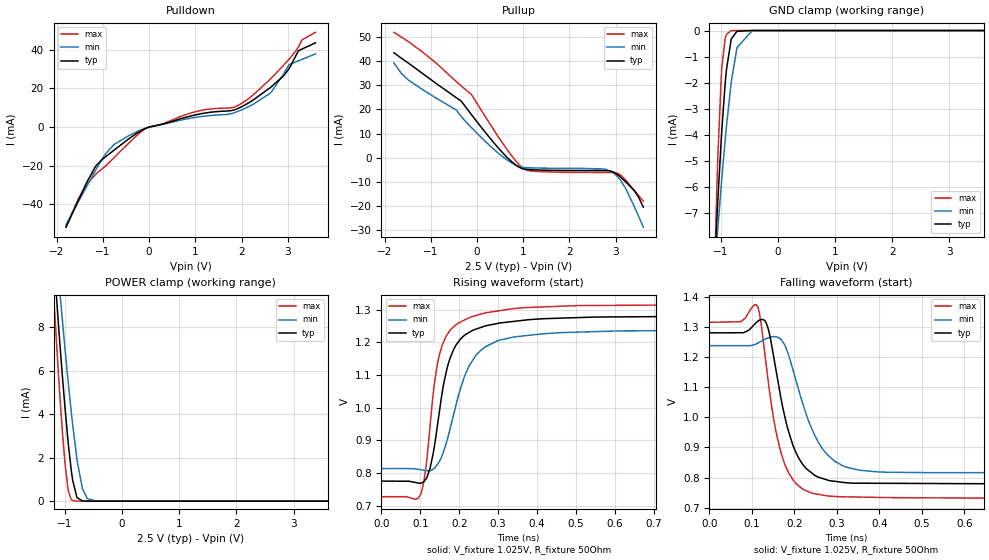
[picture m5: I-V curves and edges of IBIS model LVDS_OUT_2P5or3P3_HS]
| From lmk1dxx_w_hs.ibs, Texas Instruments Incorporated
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|   LVDS_OUT_2P5or3P3_HS Model
[Model]   LVDS_OUT_2P5or3P3_HS
Model_type   Output
Polarity   Non-Inverting
Vmeas = 1.025
Vref = 1.025
Cref = 2pF
Rref = 50
|   typ   min   max
C_comp   0.89pF   0.82pF   0.98pF
[Rac]   50   NA   NA
[Cac]   2p   NA   NA
[Voltage Range]   2.5   2.375   2.625
[Temperature Range]   45   150   -40
[Pullup Reference]   2.5   2.375   2.625
[Pulldown Reference]   0   0   0
[Power Clamp Reference]   2.5   2.375   2.625
[GND Clamp Reference]   0   0   0
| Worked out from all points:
|   slope of the pulldown table from 0 to 0.375 V, typ, clamps not added: 182 ohm
|   slope of the pullup table from 0 to 0.375 V, typ, clamps not added: 41.9 ohm
|   GND clamp passes 1 mA (typ) near -0.87 V on its own axis
|   POWER clamp passes 1 mA (typ) near -0.87 V on its own axis
|   falling waveform, V_fixture 1.025V, R_fixture 50Ohm: 20-80 % time 52.4ps typ, 67.7ps min, 45.7ps max; typ from 1.28 V to 0.775 V
|   rising waveform, V_fixture 1.025V, R_fixture 50Ohm: 20-80 % time 51ps typ, 70.8ps min, 41.6ps max; typ from 0.775 V to 1.28 V
[Pulldown]
|   Voltage   I(typ)   I(min)   I(max)
-1.8V     -51.71mA   -50.46mA   -51.59mA
-1.532V   -37.86mA   -38.59mA   -36.99mA
-1.175V   -20.92mA   -22.95mA   -24.82mA
-763.7mV  -11.99mA   -9.059mA   -15.94mA
-42.3mV   -331.8uA   -287uA     -398.5uA
1.007V    6.329mA    5.035mA    7.964mA
2.004V    10.56mA    8.93mA     12.31mA
2.61V     20.21mA    17.33mA    24.49mA
3.028V    30.21mA    32.21mA    35.05mA
3.232V    39.43mA    34.24mA    41.46mA
3.307V    40.33mA    34.98mA    45.04mA
3.6V      43.54mA    37.85mA    48.98mA
[GND Clamp]
|   Voltage   I(typ)   I(min)   I(max)
-1.8V     -47.22mA   -32.28mA   -90.43mA
-1.103V   -8.782mA   -9.069mA   -8.722mA
-1.072V   -7.372mA   -8.153mA   -6.225mA
-1.053V   -6.556mA   -7.61mA    -4.893mA
-988.9mV  -4.055mA   -5.855mA   -1.636mA
-982.4mV  -3.827mA   -5.684mA   -1.42mA
-922.5mV  -2.008mA   -4.177mA   -294.7uA
-899.8mV  -1.477mA   -3.648mA   -144.9uA
-818.3mV  -346uA     -1.998mA   -5.222uA
-717.3mV  -29.3uA    -659.5uA   -36.6nA
-450mV    -2.386nA   -3.724uA   -6.465pA
3.6V      0A         0A         0A
[Pullup]
|   Voltage   I(typ)   I(min)   I(max)
-1.8V     43.62mA    39.39mA    52.14mA
-1.481V   39.25mA    32.16mA    48.18mA
-450mV    24.91mA    19.81mA    31.63mA
-347.4mV  23.58mA    17.22mA    29.89mA
-122.2mV  17.9mA     12.47mA    26.28mA
581.9mV   1.41mA     -27.44uA   5.168mA
1.007V    -4.767mA   -4.124mA   -4.59mA
1.39V     -5.227mA   -4.407mA   -5.881mA
2.89V     -5.648mA   -5.748mA   -6.237mA
3.15V     -8.931mA   -10.75mA   -8.061mA
3.399V    -13.74mA   -20.23mA   -13.55mA
3.6V      -20.68mA   -29.01mA   -18.2mA
[POWER Clamp]
|   Voltage   I(typ)   I(min)   I(max)
-1.8V     35.35mA    33.02mA    38.41mA
-1.235V   12.58mA    14.14mA    11.07mA
-1.108V   7.901mA    10.18mA    5.58mA
-1.068V   6.535mA    8.999mA    4.045mA
-1V       4.324mA    7.032mA    1.764mA
-945.7mV  2.747mA    5.536mA    547.3uA
-890.1mV  1.424mA    4.11mA     81.35uA
-863.6mV  938uA      3.477mA    28.21uA
-793.4mV  199.1uA    1.989mA    1.463uA
-694.6mV  11.18uA    577.1uA    13.83nA
-607.7mV  708.9nA    109.9uA    194.5pA
3.6V      0A         0A         0A
[Ramp]
R_load = 50
|   typ   min   max
dV/dt_r   0.303343/5.09985e-11   0.254874/7.05739e-11   0.352823/4.14866e-11
dV/dt_f   0.303553/5.23312e-11   0.2554/6.74673e-11   0.352879/4.57533e-11
[Falling Waveform]
V_fixture = 1.025V
V_fixture_min = 1.025V
V_fixture_max = 1.025V
R_fixture = 50Ohm
C_fixture = 0F
|   Time   V(typ)   V(min)   V(max)
0s        1.281V     1.238V     1.316V
73.22ps   1.281V     1.238V     1.317V
112.9ps   1.318V     1.246V     1.37V
137.3ps   1.3V       1.263V     1.134V
156.8ps   1.158V     1.268V     953.8mV
177.7ps   1.002V     1.239V     844.3mV
215.8ps   852.2mV    1.064V     766.3mV
279.8ps   791mV      873.2mV    738.8mV
521.3ps   780.3mV    816.3mV    732.7mV
5ns       774.8mV    812.5mV    727.8mV
[Rising Waveform]
V_fixture = 1.025V
V_fixture_min = 1.025V
V_fixture_max = 1.025V
R_fixture = 50Ohm
C_fixture = 0F
|   Time   V(typ)   V(min)   V(max)
0s        775.4mV    813.9mV    727.8mV
100.6ps   768.9mV    810.6mV    734.9mV
114.4ps   781.5mV    807.7mV    818.2mV
124.9ps   814.6mV    807.8mV    943.4mV
142ps     929.4mV    823.5mV    1.121V
173ps     1.139V     919.5mV    1.231V
211.5ps   1.219V     1.089V     1.267V
240.5ps   1.239V     1.156V     1.281V
335.7ps   1.264V     1.215V     1.303V
5ns       1.281V     1.239V     1.316V
